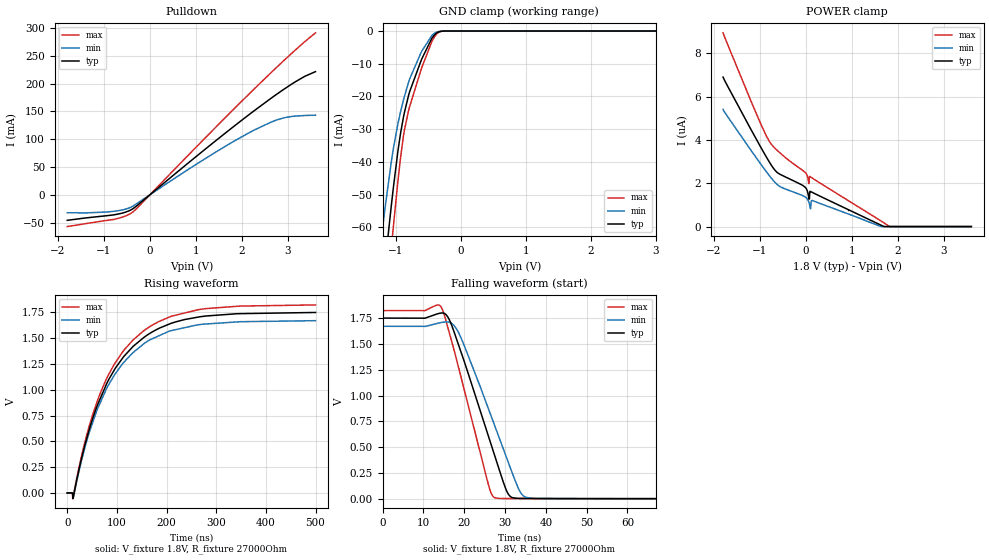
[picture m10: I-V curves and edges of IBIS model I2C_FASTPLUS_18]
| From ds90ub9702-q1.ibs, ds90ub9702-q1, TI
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|   I2C_FastPlus18 Model
[Model]   I2C_FASTPLUS_18
Model_type   I/O_open_drain
Polarity   Non-Inverting
Enable   Active-High
Vinl = 0.54
Vinh = 1.26
Vmeas = 0.9
Vref = 1.8
Cref = 0pF
Rref = 27000
|   typ   min   max
C_comp   1.3293528pF  1.3920023pF  1.3293528pF
[Voltage Range]   1.8   1.71   1.89
[Temperature Range]   27   105   -40
[Pullup Reference]   1.8   1.71   1.89
[Pulldown Reference]   0   0   0
[Power Clamp Reference]   1.8   1.71   1.89
[GND Clamp Reference]   0   0   0
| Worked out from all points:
|   slope of the pulldown table from 0 to 0.27 V, typ, clamps not added: 14.5 ohm
|   GND clamp passes 1 mA (typ) near -0.39 V on its own axis
|   falling waveform, V_fixture 1.8V, R_fixture 27000Ohm: 20-80 % time 8.62ns typ, 9.52ns min, 7.06ns max; typ from 1.75 V to 0.001 V
|   rising waveform, V_fixture 1.8V, R_fixture 27000Ohm: 20-80 % time 99ns typ, 97.7ns min, 98.8ns max; typ from 0.001 V to 1.75 V
[Pulldown]
|   Voltage   I(typ)   I(min)   I(max)
-1.8V     -46.05mA   -32.39mA   -57.33mA
-1.39V    -41.67mA   -32.67mA   -51.89mA
-801mV    -36.39mA   -29.97mA   -44.68mA
-531mV    -31.37mA   -25.98mA   -38.26mA
-369mV    -25.03mA   -20.3mA    -30.81mA
1.219V    83.16mA    65.87mA    103.7mA
1.796V    121.2mA    94.83mA    151.9mA
2.266V    151.2mA    116.4mA    190.4mA
2.628V    173.3mA    130.5mA    219.4mA
2.909V    189.7mA    138.3mA    241.3mA
3.357V    212.7mA    142.6mA    274.8mA
3.6V      221.6mA    143.2mA    291.5mA
[GND Clamp]
|   Voltage   I(typ)   I(min)   I(max)
-1.8V     -199.4mA   -169.6mA   -233.1mA
-1.217V   -81.45mA   -62.71mA   -99.08mA
-1.195V   -77.25mA   -59.17mA   -94.26mA
-1.163V   -71.03mA   -53.98mA   -87.07mA
-1.071V   -54.02mA   -40.47mA   -67.16mA
-1.039V   -48.35mA   -36.29mA   -60.36mA
-919.8mV  -30.64mA   -24.24mA   -37.84mA
-865.8mV  -24.89mA   -19.99mA   -30.25mA
-801mV    -19.58mA   -15.58mA   -24.22mA
-595.8mV  -8.39mA    -6.051mA   -11mA
-390.6mV  -916.2uA   -527.9uA   -1.415mA
3.6V      0A         0A         0A
[POWER Clamp]
|   Voltage   I(typ)   I(min)   I(max)
-1.8V     6.905uA    5.414uA    8.951uA
-790.2mV  2.974uA    2.348uA    3.928uA
-606.6mV  2.475uA    1.914uA    3.491uA
-12.6mV   1.815uA    1.368uA    2.501uA
36mV      1.629uA    1.267uA    2.314uA
68.4mV    1.266uA    1.118uA    1.987uA
79.2mV    1.285uA    1.038uA    2.319uA
84.6mV    1.557uA    989.8nA    2.319uA
100.8mV   1.623uA    827nA      2.295uA
133.2mV   1.587uA    1.209uA    2.25uA
1.818V    0A         0A         1.266nA
3.6V      0A         0A         0A
[Ramp]
R_load = 27000
|   typ   min   max
dV/dt_r   1.04924/9.87485e-08   1.00136/9.7326e-08   1.09317/9.84665e-08
dV/dt_f   1.05035/8.62189e-09   1.00256/9.51609e-09   1.0941/7.05487e-09
[Falling Waveform]
V_fixture = 1.8V
V_fixture_min = 1.71V
V_fixture_max = 1.89V
R_fixture = 27000Ohm
C_fixture = 0F
|   Time   V(typ)   V(min)   V(max)
0s        1.752V     1.672V     1.824V
14.4ns    1.801V     1.709V     1.854V
16.3ns    1.738V     1.711V     1.614V
18.68ns   1.482V     1.605V     1.26V
26.24ns   567.2mV    838mV      92.11mV
28.34ns   309.7mV    614.1mV    3.969mV
30.79ns   45.16mV    353mV      2.775mV
33.75ns   3.357mV    64.12mV    2.466mV
37.64ns   1.877mV    4.343mV    2.059mV
500ns     961.3uV    1.134mV    814.6uV
[Rising Waveform]
V_fixture = 1.8V
V_fixture_min = 1.71V
V_fixture_max = 1.89V
R_fixture = 27000Ohm
C_fixture = 0F
|   Time   V(typ)   V(min)   V(max)
0s        961.3uV    1.134mV    814.6uV
10.17ns   950.1uV    1.124mV    813.8uV
11.25ns   -43.03mV   -8.063mV   -55.06mV
12.3ns    -38.58mV   -46.24mV   -29.75mV
41.97ns   575mV      547.1mV    608.1mV
77.9ns    1.042V     998.3mV    1.094V
112.1ns   1.311V     1.256V     1.37V
153.2ns   1.503V     1.442V     1.569V
264.8ns   1.706V     1.631V     1.778V
500ns     1.75V      1.67V      1.823V
